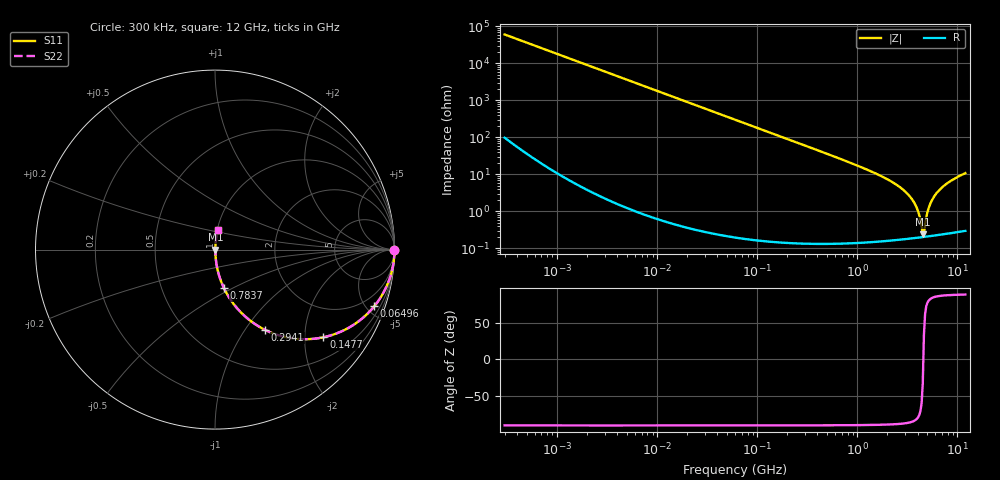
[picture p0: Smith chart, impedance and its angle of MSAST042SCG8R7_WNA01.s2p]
! MSAST042SCG8R7_WNA01  S-PARAMETER MODEL  ( General Type )
! Model Generated by TAIYO YUDEN Corporation (http://www.ty-top.com)
! Version 1.0
! TAIYO YUDEN Control No. 150820
! Copyright(c) 2015 TAIYO YUDEN CO.,LTD. All Rights Reserved.
! Product Description (link to TY-COMPAS)
! https://ds.yuden.co.jp/TYCOMPAS/or/detail?pn=MSAST042SCG8R7BWNA01&u=M
! Products Name : Multilayer Ceramic Capacitors
! Characteristics :
!  Capacitance : 8.7 pF , Rated Voltage : 25V , TCC : CG / C0G
!  Case Size : 0.4 x 0.2 / 0.016 x 0.008 [mm/inch] , Thickness : 0.2 / 0.008 [mm/inch]
!  (Conditions: Temperature = 25 degC , DC Bias Current/Voltage = 0A / 0V)
! External Node Assignments :
!  1  o---| |---o  2
! GND o---------o GND
! Frequency Range : 0.3MHz  -  12000MHz  [ 401 STEP ]
# MHz S RI R 50
! Freq[MHz].  S11 Real  S11 Imag  S21 Real  S21 Imag  S12 Real  S12 Imag  S22 Real  S22 Imag
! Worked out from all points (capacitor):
!   401 points, 300 kHz to 12 GHz, reference 50 ohm
!   read as one part in series: C = 8.72 pF near 316.3 kHz
!   lowest |Z| = 241 mohm at 4.503 GHz (marker M1)
!   series resonance near 4.562 GHz, so ESL is about 140 pH
!   S11 on the Smith chart (normalised r, x): 300 kHz: open; 64.96 MHz: 1.00, -5.62; 147.7 MHz: 1.00, -2.47; 294.1 MHz: 1.00, -1.24; 783.7 MHz: 1.00, -0.45; 12 GHz: 1.01, +0.22
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0.3  1 -0.00164  5.37e-06 0.00164  5.37e-06 0.00164  1 -0.00164
1.769972  0.9999 -0.00969  9.82e-05 0.00969  9.82e-05 0.00969  0.9999 -0.00969
10.44266  0.9967 -0.057  0.00328 0.057  0.00328 0.057  0.9967 -0.057
26.39317  0.9795 -0.1416  0.0205 0.1416  0.0205 0.1416  0.9795 -0.1416
60  0.9023 -0.2965  0.0977 0.2965  0.0977 0.2965  0.9023 -0.2965
64.96309  0.8874 -0.3157  0.1126 0.3157  0.1126 0.3157  0.8874 -0.3157
147.6816  0.6039 -0.4885  0.3961 0.4885  0.3961 0.4885  0.6039 -0.4885
294.0765  0.277 -0.4464  0.723 0.4464  0.723 0.4464  0.277 -0.4464
353.9943  0.2087 -0.4051  0.7913 0.4051  0.7913 0.4051  0.2087 -0.4051
783.7017  0.0498 -0.2146  0.9502 0.2146  0.9502 0.2146  0.0498 -0.2146
2088.533  0.00636 -0.0687  0.9936 0.0687  0.9936 0.0687  0.00636 -0.0687
2795.104  0.00341 -0.0408  0.9966 0.0408  0.9966 0.0408  0.00341 -0.0408
3454.93  0.00237 -0.0227  0.9976 0.0227  0.9976 0.0227  0.00237 -0.0227
3944.255  0.00208 -0.0119  0.9979 0.0119  0.9979 0.0119  0.00208 -0.0119
4385.161  0.00202 -0.00342  0.998 0.00342  0.998 0.00342  0.00202 -0.00342
4502.883  0.00203 -0.0013  0.998 0.0013  0.998 0.0013  0.00203 -0.0013
4747.894  0.00208 0.00383  0.9979 -0.00383  0.9979 -0.00383  0.00208 0.00383
5006.236  0.00219 0.00916  0.9978 -0.00916  0.9978 -0.00916  0.00219 0.00916
5278.635  0.00235 0.0145  0.9976 -0.0145  0.9976 -0.0145  0.00235 0.0145
6188.031  0.00325 0.0312  0.9968 -0.0312  0.9968 -0.0312  0.00325 0.0312
8064.993  0.00608 0.0595  0.9939 -0.0595  0.9939 -0.0595  0.00608 0.0595
12000  0.0146 0.1068  0.9854 -0.1068  0.9854 -0.1068  0.0146 0.1068
